// Implicitly generated code : DO NOT EDIT
FUNCTION CheckBounds : DINT
VAR_INPUT
	index, lower, upper: DINT;
END_VAR

// Implicitly generated code : Only an Implementation suggestion
IF  index < lower THEN
	CheckBounds := lower;
	giCheckUnder := giCheckUnder +1; 
ELSIF  index > upper THEN
	CheckBounds := upper;
	giCheckOver:= giCheckOver +1; 
ELSE  
	CheckBounds := index;
END_IF

END_FUNCTION
